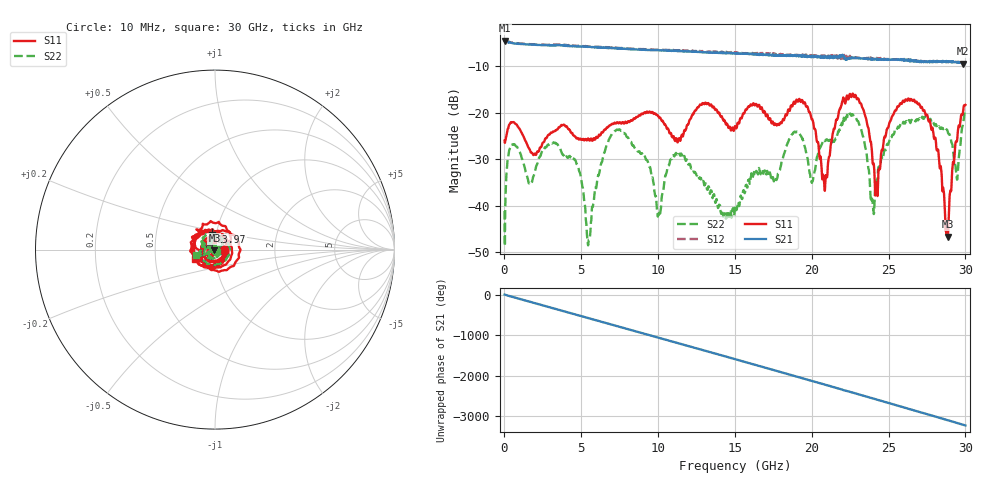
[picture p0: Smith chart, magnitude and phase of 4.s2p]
!Agilent Technologies,E8364B,US42250130,A.04.87.01
!Agilent E8364B: A.04.87.01
!Date: Monday, February 07, 2022 23:46:52
!Correction: S11(Full 2 Port SOLT,1,2) S21(Full 2 Port SOLT,1,2) S12(Full 2 Port SOLT,1,2) S22(Full 2 Port SOLT,1,2)
!S2P File: Measurements: S11, S21, S12, S22:
# Hz S  dB  R 50
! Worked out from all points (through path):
!   1601 points, 10 MHz to 30 GHz, reference 50 ohm
!   highest |S21| = -4.50 dB at 28.74 MHz (marker M1); lowest = -9.5 dB at 29.85 GHz (marker M2)
!   group delay of S21, straight-line fit = 298 ps
!   lowest |S11| = -46.7 dB at 28.86 GHz (marker M3), VSWR 1.01, Z = 49.7 - j0.355 ohm
!   |S11| at or under -10 dB: start of sweep to end of sweep
!   |S22| runs from -48.7 to -19.4 dB; largest |S21 - S12| = 0.056
!   S11 on the Smith chart (normalised r, x): 10 MHz: 1.11, -0.01; 13.97 GHz: 0.95, +0.19; 30 GHz: 0.80, -0.08
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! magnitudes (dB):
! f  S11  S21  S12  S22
! 10 MHz  -26.0  -4.6  -4.6  -41.1
! 28.74 MHz  -26.5  -4.5  -4.5  -48.7
! 553.6 MHz  -22.0  -5.0  -4.9  -26.9
! 5.015 GHz  -25.8  -5.8  -5.7  -34.7
! 5.502 GHz  -25.8  -5.9  -5.7  -47.3
! 7.564 GHz  -22.2  -6.2  -6.1  -23.9
! 10.02 GHz  -20.8  -6.6  -6.5  -41.9
! 11.24 GHz  -26.0  -6.7  -6.6  -29.0
! 13.97 GHz  -20.0  -7.1  -6.9  -39.8
! 15.01 GHz  -22.9  -7.2  -7.2  -40.6
! 18.9 GHz  -18.1  -7.8  -7.7  -24.1
! 20.01 GHz  -21.3  -7.8  -7.6  -35.1
! 20.85 GHz  -36.8  -8.2  -7.7  -26.0
! 22.93 GHz  -17.1  -8.3  -8.2  -21.5
! 23.95 GHz  -29.8  -8.4  -8.3  -38.6
! 24.23 GHz  -35.7  -8.5  -8.2  -34.9
! 25.01 GHz  -22.7  -8.6  -8.5  -26.4
! 27.39 GHz  -20.3  -9.1  -8.9  -21.1
! 28.86 GHz  -46.7  -8.9  -9.0  -24.1
! 29.42 GHz  -26.3  -9.1  -9.2  -33.5
! 29.85 GHz  -19.7  -9.5  -9.2  -22.3
! 30 GHz  -18.3  -9.2  -9.3  -19.4
